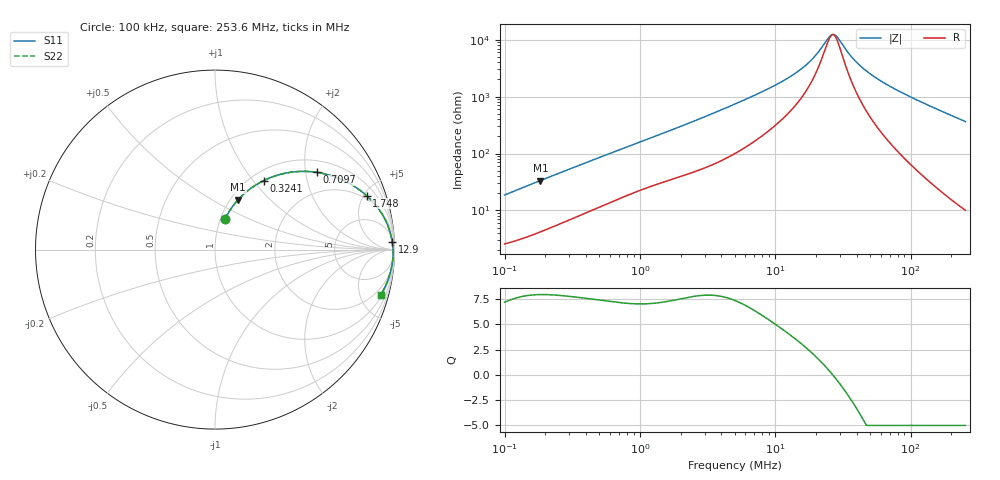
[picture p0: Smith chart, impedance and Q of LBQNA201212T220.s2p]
! LBQNA201212T220  S-PARAMETER MODEL  ( General Type )
! Model Generated by TAIYO YUDEN Corporation (http://www.ty-top.com)
! Version 1.0
! TAIYO YUDEN Control No. 191025NI43SB-FBB
! Copyright(c) 2019 TAIYO YUDEN CO.,LTD. All Rights Reserved.
! Product Description (link to TY-COMPAS)
! https://ds.yuden.co.jp/TYCOMPAS/or/detail?pn=LBQNA201212T220K&u=M
! Products Name : Inductors
! Characteristics :
!  Inductance : 22 uH , SRF(min) : 16 MHz , DC Resistance(max) : 2.21 Ohm
!  Rated Current : Saturation :135 mA , Temp Rise : 220 mA (20 degC)
!  Case Size : 2.0 x 1.25 / 0.079 x 0.049 [mm/inch] , Thickness : 1.25 / 0.049 [mm/inch]
!  (Conditions: Temperature = 25 degC , DC Bias Current/Voltage = 0A / 0V)
! External Node Assignments :
!  1  o---GGG---o  2
! GND o---------o GND
! Frequency Range : 0.1MHz  -  253.640152MHz  [ 402 STEP ]
# MHz S RI R 50
! Freq[MHz].  S11 Real  S11 Imag  S21 Real  S21 Imag  S12 Real  S12 Imag  S22 Real  S22 Imag
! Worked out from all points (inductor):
!   401 points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, 100 kHz to 253.6 MHz, reference 50 ohm
!   read as one part in series: L = 29.2 uH near 104 kHz
!   highest Q = 7.93 at 183.6 kHz (marker M1), where L = 28.8 uH
!   self-resonance near 26.12 MHz
!   S11 on the Smith chart (normalised r, x): 100 kHz: 1.05, +0.37; 324.1 kHz: 1.15, +1.13; 709.7 kHz: 1.32, +2.32; 1.748 MHz: 1.71, +5.24; 12.9 MHz: 12, +44; 253.6 MHz: 1.20, -7.29
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0.1  0.0558 0.1702  0.9442 -0.1702  0.9442 -0.1702  0.0558 0.1702
0.183581  0.1286 0.2776  0.8714 -0.2776  0.8714 -0.2776  0.1286 0.2776
0.324065  0.2704 0.384  0.7296 -0.384  0.7296 -0.384  0.2704 0.384
0.371712  0.3167 0.4041  0.6833 -0.4041  0.6833 -0.4041  0.3167 0.4041
0.709667  0.5682 0.4302  0.4318 -0.4302  0.4318 -0.4302  0.5682 0.4302
1.381698  0.789 0.3438  0.211 -0.3438  0.211 -0.3438  0.789 0.3438
1.747993  0.8443 0.3009  0.1557 -0.3009  0.1557 -0.3009  0.8443 0.3009
2.853009  0.9224 0.2113  0.0776 -0.2113  0.0776 -0.2113  0.9224 0.2113
5.03627  0.9655 0.1267  0.0345 -0.1267  0.0345 -0.1267  0.9655 0.1267
8.717747  0.9819 0.0707  0.0181 -0.0707  0.0181 -0.0707  0.9819 0.0707
12.90076  0.9874 0.042  0.0126 -0.042  0.0126 -0.042  0.9874 0.042
15.69353  0.9892 0.0298  0.0108 -0.0298  0.0108 -0.0298  0.9892 0.0298
18.72042  0.9904 0.0195  0.00958 -0.0195  0.00958 -0.0195  0.9904 0.0195
25.11734  0.9918 0.00311  0.0082 -0.00311  0.0082 -0.00311  0.9918 0.00311
27.16539  0.992 -0.00126  0.00796 0.00126  0.00796 0.00126  0.992 -0.00126
28.81028  0.9922 -0.00455  0.00783 0.00455  0.00783 0.00455  0.9922 -0.00455
35.04717  0.9924 -0.0158  0.00762 0.0158  0.00762 0.0158  0.9924 -0.0158
41.80689  0.9922 -0.0265  0.00778 0.0265  0.00778 0.0265  0.9922 -0.0265
51.86374  0.9915 -0.0409  0.0085 0.0409  0.0085 0.0409  0.9915 -0.0409
69.58603  0.9893 -0.0636  0.0107 0.0636  0.0107 0.0636  0.9893 -0.0636
125.2675  0.977 -0.1267  0.023 0.1267  0.023 0.1267  0.977 -0.1267
253.6402  0.9241 -0.2514  0.0759 0.2514  0.0759 0.2514  0.9241 -0.2514
